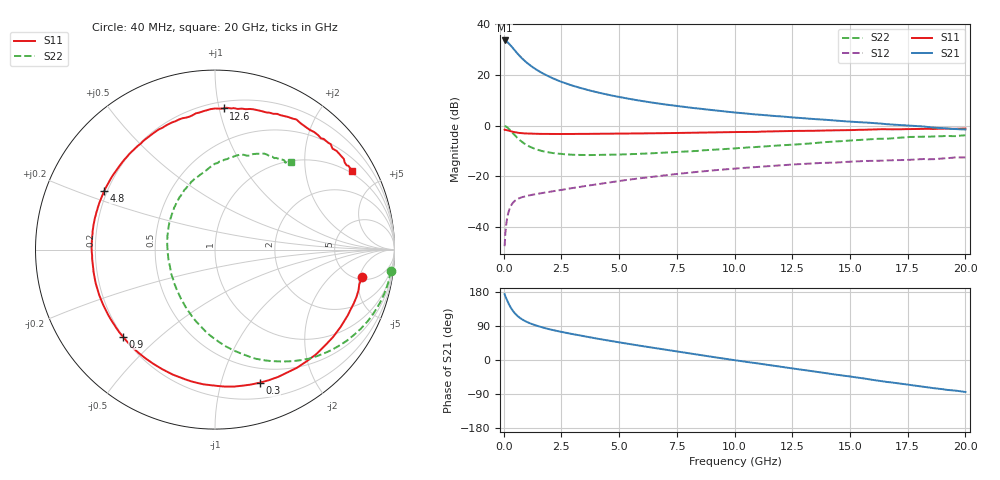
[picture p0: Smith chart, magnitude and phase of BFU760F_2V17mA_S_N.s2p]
! Filename:  P:\Prog\Test\Noise\ATS_data\Testdata_Net\BFU760\BFU760F_2W_C1_2V17mA_D.s2p
! Date/Time: Mon 06/Feb/2012 15:05:34
! BFU760_2W_C1_2V17mA
! bias mode 1: Vout= 2.0003 V, Iout=17.0300 mA, Vin= 0.7843 V, Iin= 0.0524 mA
! Date/time Fri Mar 18 14:16:23 2011
! Device data file deembeded for feedlines and parallel
! Original file: \BFU760\BFU760_2W_C1_2V17mA_R.s2p
! Feed-files: PR003V01_101208_Feed1.s2p, PR003V01_101208_Feed2.s2p
! Parallel-file: PR003V01_101208_Par.s2p
# MHz S MA R 50
!  Freq-MHz  S11-mag  S11-arg  S21-mag  S21-arg  S12-mag  S12-arg  S22-mag  S22-arg
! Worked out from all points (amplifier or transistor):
!   167 points, 40 MHz to 20 GHz, reference 50 ohm
!   highest |S21| = 33.7 dB at 40 MHz (marker M1)
!   |S21| within 3 dB of that: start of sweep to 397.3 MHz
!   unconditionally stable (mu >= 1): 4.541 GHz to 13.72 GHz
!   at 550 MHz: K = 0.21, MSG = 29.1 dB, |S12| = -29.2 dB
!   at 4.2 GHz: K = 0.98, MSG = 17.9 dB, |S12| = -22.9 dB
!   at 20 GHz: K = 0.88, MSG = 5.5 dB, |S12| = -12.5 dB
!   lowest NFmin = 0.48 dB at 400 MHz
!   S11 on the Smith chart (normalised r, x): 40 MHz: 5.38, -5.49; 300 MHz: 0.35, -1.33; 900 MHz: 0.20, -0.38; 4.8 GHz: 0.19, +0.24; 12.6 GHz: 0.25, +1.03; 20 GHz: 0.90, +3.52
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40  0.8344 -10.7  48.37 173.7  0.004184 82.8  0.9868 -7.0
50  0.8267 -13.6  48.26 171.6  0.004866 80.3  0.984 -9.0
90  0.8259 -23.9  47.34 165.7  0.009259 77.9  0.9704 -16.2
160  0.8131 -41.3  44.65 155.7  0.01573 69.8  0.9248 -28.4
240  0.7944 -59.6  41.42 145.5  0.02187 61.8  0.8562 -40.9
300  0.7825 -71.4  38.39 138.9  0.02552 56.6  0.802 -49.3
400  0.7598 -89.0  34.12 129.6  0.03011 49.8  0.7108 -61.1
480  0.7461 -100.1  30.75 123.5  0.03279 45.5  0.6502 -69.4
550  0.7351 -108.6  28.29 118.9  0.03451 42.7  0.5993 -75.6
700  0.7189 -122.8  23.71 111.3  0.03744 38.3  0.519 -87.0
900  0.706 -136.6  19.32 103.6  0.04006 35.0  0.4427 -99.1
1300  0.6946 -154.2  13.91 93.2  0.04387 32.4  0.357 -117.6
1850  0.6881 -169.0  9.935 83.1  0.0484 32.1  0.3033 -135.9
2500  0.6875 179.4  7.373 74.2  0.05408 33.1  0.2781 -151.8
3400  0.6907 167.4  5.454 63.6  0.06312 33.5  0.2652 -167.6
4800  0.6985 152.0  3.858 48.6  0.07875 32.0  0.2687 173.1
6800  0.7128 133.5  2.712 29.1  0.1027 26.0  0.2917 151.4
10200  0.7524 105.4  1.797 -2.2  0.1445 9.5  0.3633 120.5
12600  0.7879 86.5  1.45 -23.0  0.1725 -4.4  0.4257 101.0
13400  0.7937 80.9  1.361 -29.8  0.1812 -10.1  0.4519 94.9
16800  0.8498 54.8  1.056 -59.2  0.2075 -31.4  0.5625 69.1
20000  0.8808 30.0  0.8462 -84.4  0.2367 -53.1  0.6462 49.3
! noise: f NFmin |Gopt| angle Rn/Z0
400  0.4834  0.04525  124.8  0.0518
650  0.4854  0.08336  126.2  0.0514
1050  0.4912  0.1359  131.2  0.0503
1450  0.5001  0.1804  137.2  0.0488
1850  0.512  0.2191  143.6  0.0471
2300  0.5292  0.2585  151.3  0.0451
2900  0.5582  0.3082  161.6  0.0423
3700  0.6076  0.3738  174.4  0.0391
4500  0.6694  0.4378  185.7  0.0373
6000  0.8187  0.523  202.3  0.0401
